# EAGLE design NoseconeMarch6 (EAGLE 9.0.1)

## Sheet 1 of 3: Board to Board Headers
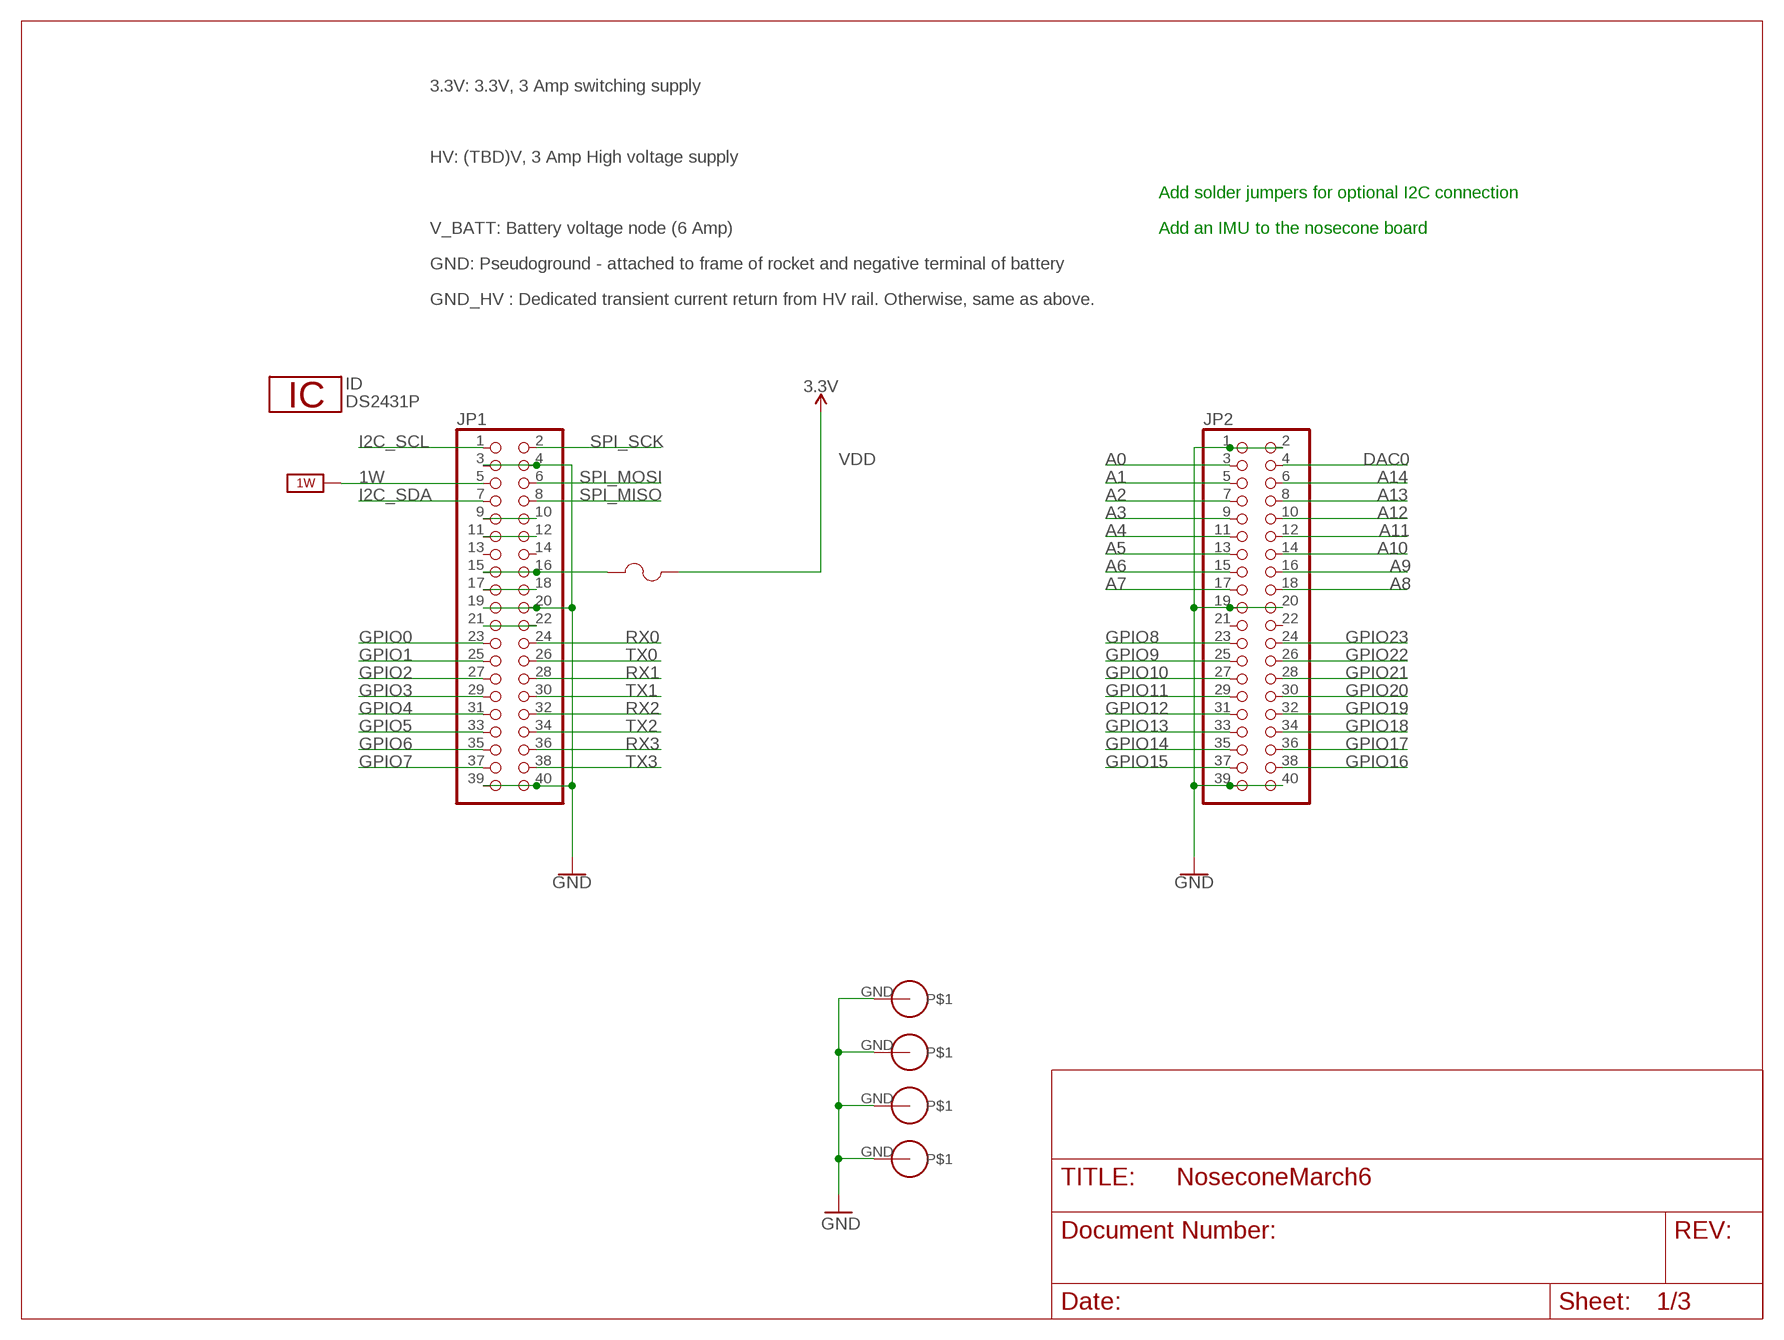
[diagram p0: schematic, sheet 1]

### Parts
F3  0603SFF150F/32-2  [FUS0603_TYCO]
ID  DS2431P  [TSOC6]
JP1  PINHD-2X20  [2X20]
JP2  PINHD-2X20  [2X20]
U$1  PS/104-MOUNTING-HOLE  [PC/104-MOUNTING-HOLE]
U$2  PS/104-MOUNTING-HOLE  [PC/104-MOUNTING-HOLE]
U$3  PS/104-MOUNTING-HOLE  [PC/104-MOUNTING-HOLE]
U$4  PS/104-MOUNTING-HOLE  [PC/104-MOUNTING-HOLE]

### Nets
1W: JP1.5 ; supply symbol labelled 1W_SUP
A0: JP2.3
A1: JP2.5
A2: JP2.7
A3: JP2.9
A4: JP2.11
A5: JP2.13
A6: JP2.15
A7: JP2.17
A8: JP2.18
A9: JP2.16
A10: JP2.14
A11: JP2.12
A12: JP2.10
A13: JP2.8
A14: JP2.6
DAC0: JP2.4
GND: JP1.3 JP1.4 JP1.19 JP1.20 JP1.39 JP1.40 JP2.1 JP2.2 JP2.19 JP2.20 JP2.39 JP2.40 U$1.GND U$2.GND U$3.GND U$4.GND ; also sheet 2,3
GND_HV: JP1.21 JP1.22
GPIO0: JP1.23 ; also sheet 3
GPIO1: JP1.25 ; also sheet 3
GPIO2: JP1.27
GPIO3: JP1.29
GPIO4: JP1.31 ; also sheet 3
GPIO5: JP1.33 ; also sheet 3
GPIO6: JP1.35 ; also sheet 2
GPIO7: JP1.37 ; also sheet 2
GPIO8: JP2.23
GPIO9: JP2.25
GPIO10: JP2.27
GPIO11: JP2.29
GPIO12: JP2.31
GPIO13: JP2.33
GPIO14: JP2.35
GPIO15: JP2.37
GPIO16: JP2.38
GPIO17: JP2.36
GPIO18: JP2.34
GPIO19: JP2.32
GPIO20: JP2.30
GPIO21: JP2.28
GPIO22: JP2.26 ; also sheet 2
GPIO23: JP2.24 ; also sheet 2
I2C_SCL: JP1.1 ; also sheet 2,3
I2C_SDA: JP1.7 ; also sheet 2,3
N$1: JP1.17 JP1.18
N$2: JP1.11 JP1.12
N$3: F3.1 JP1.15 JP1.16
N$4: JP1.9 JP1.10
RX0: JP1.24
RX1: JP1.28
RX2: JP1.32 ; also sheet 2
RX3: JP1.36 ; also sheet 2
SPI_MISO: JP1.8 ; also sheet 2,3
SPI_MOSI: JP1.6 ; also sheet 2,3
SPI_SCK: JP1.2 ; also sheet 2,3
TX0: JP1.26
TX1: JP1.30
TX2: JP1.34 ; also sheet 2
TX3: JP1.38 ; also sheet 2
VDD: F3.2 ; supply symbol labelled 3.3V ; also sheet 2,3
Unconnected: JP1.13 JP1.14 JP2.21 JP2.22

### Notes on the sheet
- 3.3V: 3.3V, 3 Amp switching supply
- HV: (TBD)V, 3 Amp High voltage supply
- Add solder jumpers for optional I2C connection
- V_BATT: Battery voltage node (6 Amp) | Add an IMU to the nosecone board
- GND: Pseudoground - attached to frame of rocket and negative terminal of battery
- GND_HV : Dedicated transient current return from HV rail. Otherwise, same as above.

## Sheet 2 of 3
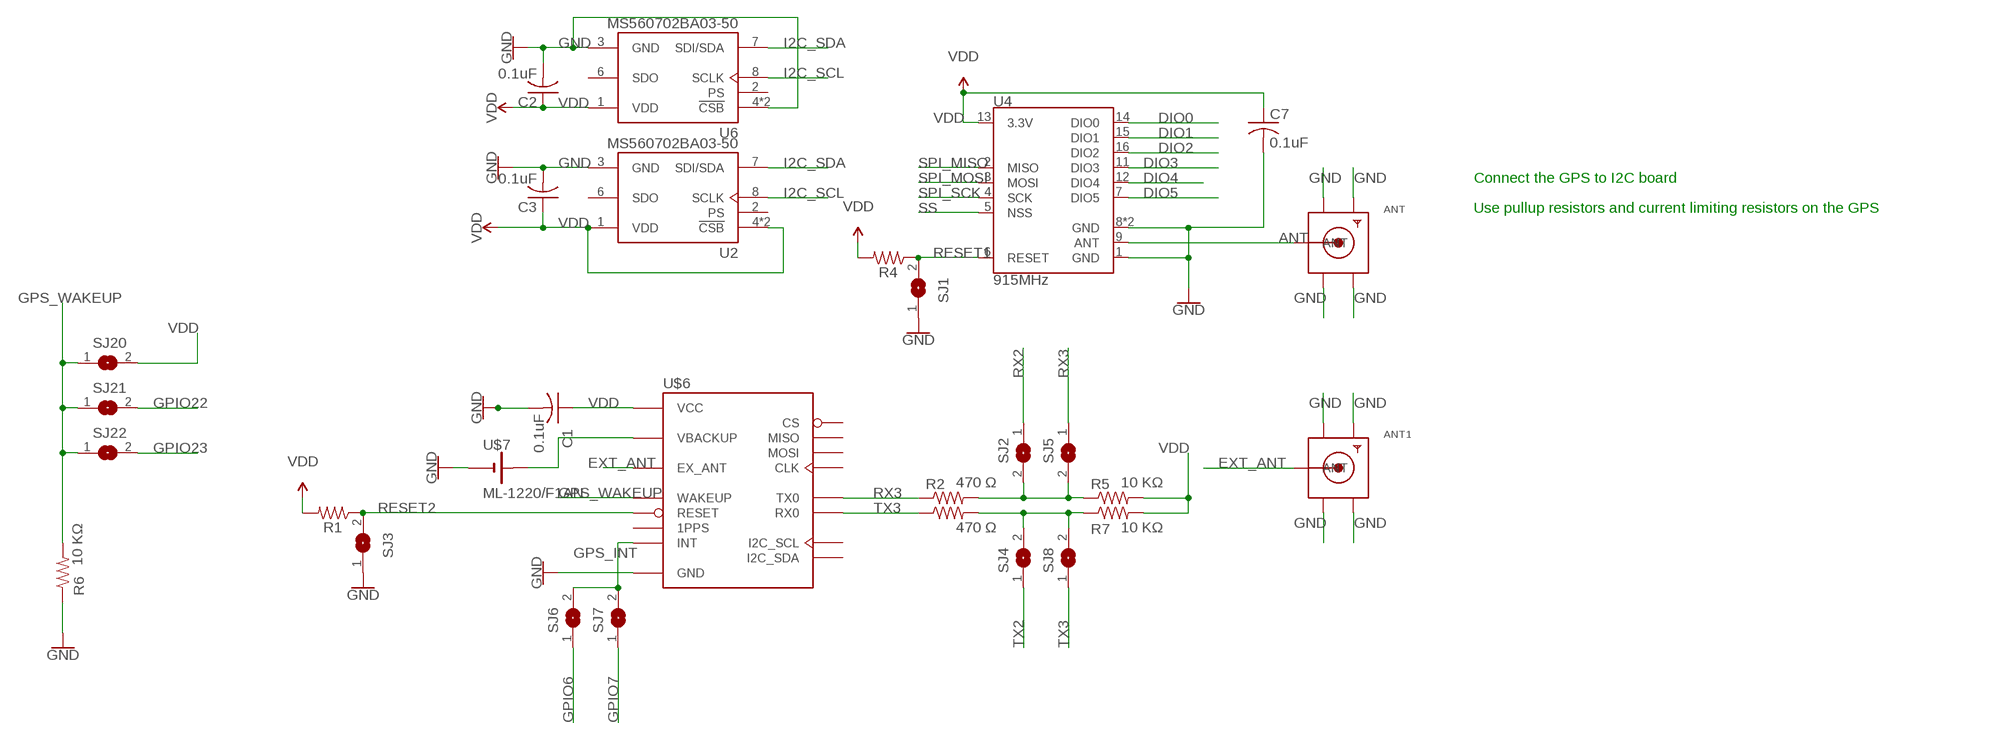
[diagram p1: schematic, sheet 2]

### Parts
ANT  SMACONNECTOR_EDGE  [SMA_EDGELAUNCH]
ANT1  SMACONNECTOR_EDGE  [SMA_EDGELAUNCH]
C1  0.1uF  C-USC0805  [C0805]
C2  0.1uF  C-USC0805  [C0805]
C3  0.1uF  C-USC0805  [C0805]
C7  0.1uF  C-USC0805  [C0805]
R1  330  R-US_R1206  [R1206]
R2  470 Ω  R-US_R1206  [R1206]
R3  470 Ω  R-US_R1206  [R1206]
R4  330  R-US_R1206  [R1206]
R5  10 KΩ  R-US_R1206  [R1206]
R6  10 KΩ  R-US_R1206  [R1206]
R7  10 KΩ  R-US_R1206  [R1206]
SJ1  SJ  [SJ]
SJ2  SJ  [SJ]
SJ3  SJ  [SJ]
SJ4  SJ  [SJ]
SJ5  SJ  [SJ]
SJ6  SJ  [SJ]
SJ7  SJ  [SJ]
SJ8  SJ  [SJ]
SJ20  SJ  [SJ]
SJ21  SJ  [SJ]
SJ22  SJ  [SJ]
U2  MS560702BA03-50  [SON125P300X500X100-8N]
U4  915MHz  RFM69HCW-915  [RFM69HCW-XXXS2]
U6  MS560702BA03-50  [SON125P300X500X100-8N]
U$6  XA1110  [XA1110]
U$7  ML-1220/F1AN  [ML-1220/F1AN]

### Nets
ANT: ANT.P(ANT) U4.9(ANT)
DIO0: U4.14(DIO0)
DIO1: U4.15(DIO1)
DIO2: U4.16(DIO2)
DIO3: U4.11(DIO3)
DIO4: U4.12(DIO4)
DIO5: U4.7(DIO5)
EXT_ANT: ANT1.P(ANT) U$6.P$2(EX_ANT)
GND: ANT1.GND@1(GND4) ANT1.GND@2(GND3) ANT1.GND@3(GND2) ANT1.GND@4(GND1) ANT.GND@1(GND4) ANT.GND@2(GND3) ANT.GND@3(GND2) ANT.GND@4(GND1) C2.2 C3.2 C7.2 R6.1 SJ1.1 SJ3.1 U2.3(GND) U4.1(GND) U4.8(GND) U4.10(GND) U6.3(GND) U6.4(!CSB) U6.5(!CSB) U$6.P$1(GND) U$6.P$3(GND) U$6.P$4(GND) U$6.P$5(GND) U$6.P$6(GND) U$6.P$9(GND) U$6.P$10(GND) U$6.P$11(GND) U$6.P$24(GND) ; also sheet 1,3
GPIO6: SJ6.1 ; also sheet 1
GPIO7: SJ7.1 ; also sheet 1
GPIO22: SJ21.2 ; also sheet 1
GPIO23: SJ22.2 ; also sheet 1
GPS_INT: SJ6.2 SJ7.2 U$6.P$16(INT)
GPS_RX: R3.2 R7.1 SJ4.2 SJ8.2
GPS_TX: R2.2 R5.1 SJ2.2 SJ5.2
GPS_WAKEUP: R6.2 SJ20.1 SJ21.1 SJ22.1 U$6.P$12(WAKEUP)
I2C_SCL: U2.8(SCLK) U6.8(SCLK) ; also sheet 1,3
I2C_SDA: U2.7(SDI/SDA) U6.7(SDI/SDA) ; also sheet 1,3
N$5: U$7.NEG(N) ; supply symbol labelled GND
N$6: C1.2
RESET1: R4.1 SJ1.2 U4.6(RESET)
RESET2: R1.1 SJ3.2 U$6.P$22(RESET)
RX2: SJ2.1 ; also sheet 1
RX3: R2.1 SJ5.1 U$6.P$19(TX0) ; also sheet 1
SPI_MISO: U4.2(MISO) ; also sheet 1,3
SPI_MOSI: U4.3(MOSI) ; also sheet 1,3
SPI_SCK: U4.4(SCK) ; also sheet 1,3
SS: U4.5(NSS)
TX2: SJ4.1 ; also sheet 1
TX3: R3.1 SJ8.1 U$6.P$20(RX0) ; also sheet 1
VBACKUP: U$6.P$8(VBACKUP) U$7.POS(P)
VDD: C1.1 C2.1 C3.1 C7.1 R1.2 R4.2 R5.2 R7.2 SJ20.2 U2.1(VDD) U2.4(!CSB) U2.5(!CSB) U4.13(3.3V) U6.1(VDD) U$6.P$7(VCC) ; also sheet 1,3
Unconnected: U2.2(PS) U2.6(SDO) U6.2(PS) U6.6(SDO) U$6.P$13(I2C_SDA) U$6.P$14(I2C_SCL) U$6.P$15(MISO) U$6.P$17(MOSI) U$6.P$18(CLK) U$6.P$21(1PPS) U$6.P$23(CS)

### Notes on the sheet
- Connect the GPS to I2C board
- Use pullup resistors and current limiting resistors on the GPS

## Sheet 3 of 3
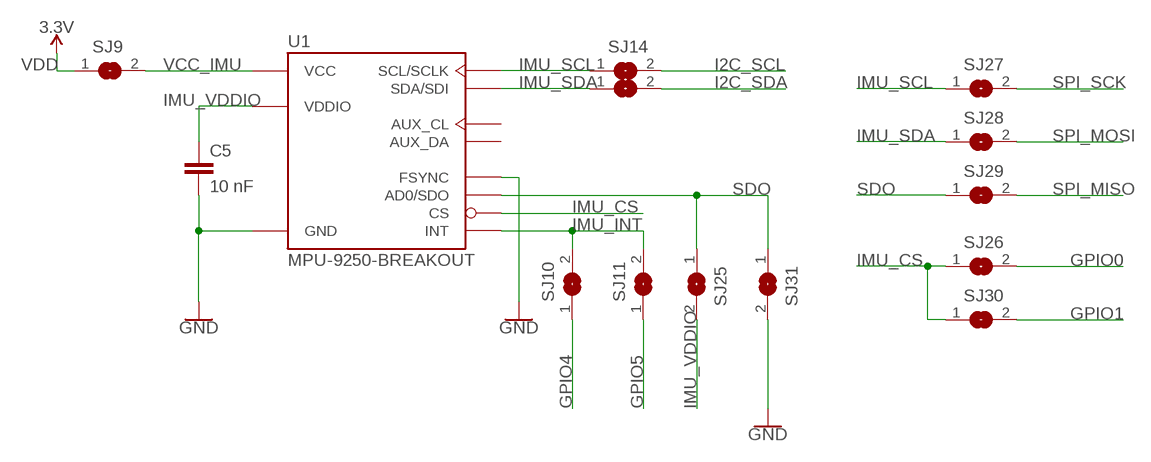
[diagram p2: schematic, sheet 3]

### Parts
C5  10 nF  C-EUC0805  [C0805]
SJ9  SJ  [SJ]
SJ10  SJ  [SJ]
SJ11  SJ  [SJ]
SJ14  SJ  [SJ]
SJ15  SJ  [SJ]
SJ25  SJ  [SJ]
SJ26  SJ  [SJ]
SJ27  SJ  [SJ]
SJ28  SJ  [SJ]
SJ29  SJ  [SJ]
SJ30  SJ  [SJ]
SJ31  SJ  [SJ]
U1  MPU-9250-BREAKOUT  [MPU-9250-BREAKOUT]

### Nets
GND: C5.2 SJ31.2 U1.FSYNC U1.GND ; also sheet 1,2
GPIO0: SJ26.2 ; also sheet 1
GPIO1: SJ30.2 ; also sheet 1
GPIO4: SJ10.1 ; also sheet 1
GPIO5: SJ11.1 ; also sheet 1
I2C_SCL: SJ14.2 ; also sheet 1,2
I2C_SDA: SJ15.2 ; also sheet 1,2
IMU_CS: SJ26.1 SJ30.1 U1.NCS(CS)
IMU_INT: SJ10.2 SJ11.2 U1.INT
IMU_SCL: SJ14.1 SJ27.1 U1.SCL/SCLK
IMU_SDA: SJ15.1 SJ28.1 U1.SDA/SDI
IMU_VDDIO: C5.1 SJ25.2 U1.VDDIO
SDO: SJ25.1 SJ29.1 SJ31.1 U1.AD0/SDO
SPI_MISO: SJ29.2 ; also sheet 1,2
SPI_MOSI: SJ28.2 ; also sheet 1,2
SPI_SCK: SJ27.2 ; also sheet 1,2
VCC_IMU: SJ9.2 U1.VDD(VCC)
VDD: SJ9.1 ; supply symbol labelled 3.3V ; also sheet 1,2
Unconnected: U1.AUX_CL U1.AUX_DA

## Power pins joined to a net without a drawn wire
1W: ID.2(1W)
GND: ID.1(GND)

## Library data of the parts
ANT ANT1 = adafruit:SMACONNECTOR: SMA Connector 90° DIP SMA Connector, 50 Ohm (4UConnector: 07259)
C1-C3 C7 = rcl:C-US: CAPACITOR, American symbol; SPICEPREFIX: C
C5 = rcl:C-EU: CAPACITOR, European symbol; SPICEPREFIX: C
F3 = CU inSpace 2019 Parts:0603SFF150F/32-2; MANUFACTURER_PART_NUMBER: 0603SFF150F322; VENDOR: Littelfuse Inc
ID = 1wire:DS2431: 1024-Bit EEPROM
JP1 JP2 = pinhead:PINHD-2X20: PIN HEADER
R1-R7 = rcl:R-US_: RESISTOR, American symbol; SPICEPREFIX: R
SJ1-SJ11 SJ14 SJ15 SJ20-SJ22 SJ25-SJ31 = jumper:SJ: SMD solder JUMPER
U1 = Sensors Board:MPU-9250-BREAKOUT
U2 U6 = MS560702BA03-50:MS560702BA03-50: BAROMETRIC PRESSURE SENSOR; AVAILABILITY: Unavailable; DESCRIPTION: MS5607-02BA03 Series 3 V 1 to 120 kPa Absolute Barometric Pressure Sensor; EU_ROHS_COMPLIANCE: Compliant; LINK: http://www.te.com/usa-en/product-MS560702BA03-50.html; MF: TE Connectivity; MP: MS560702BA03-50; PACKAGE: SMD-8 TE Connectivity; PRICE: None
U4 = SparkFun-RF:RFM69H: Hope RF RFM69H ISM Transceiver Module The RFM69H is a transceiver module capable of operation over a wide frequency range, including the 315,433,868 and 915MHz license-free ISM (Industry Scientific and Medical) frequency bands. All major RF communication parameters are programmable and most of them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; PROD_ID: IC-11997
U$1-U$4 = CU inSpace 2019 Parts:PS/104-MOUNTING-HOLE: Mounting hole for PC/104 board.
U$6 = Sensors Board:XA1110
U$7 = Sensors Board:ML-1220/F1AN

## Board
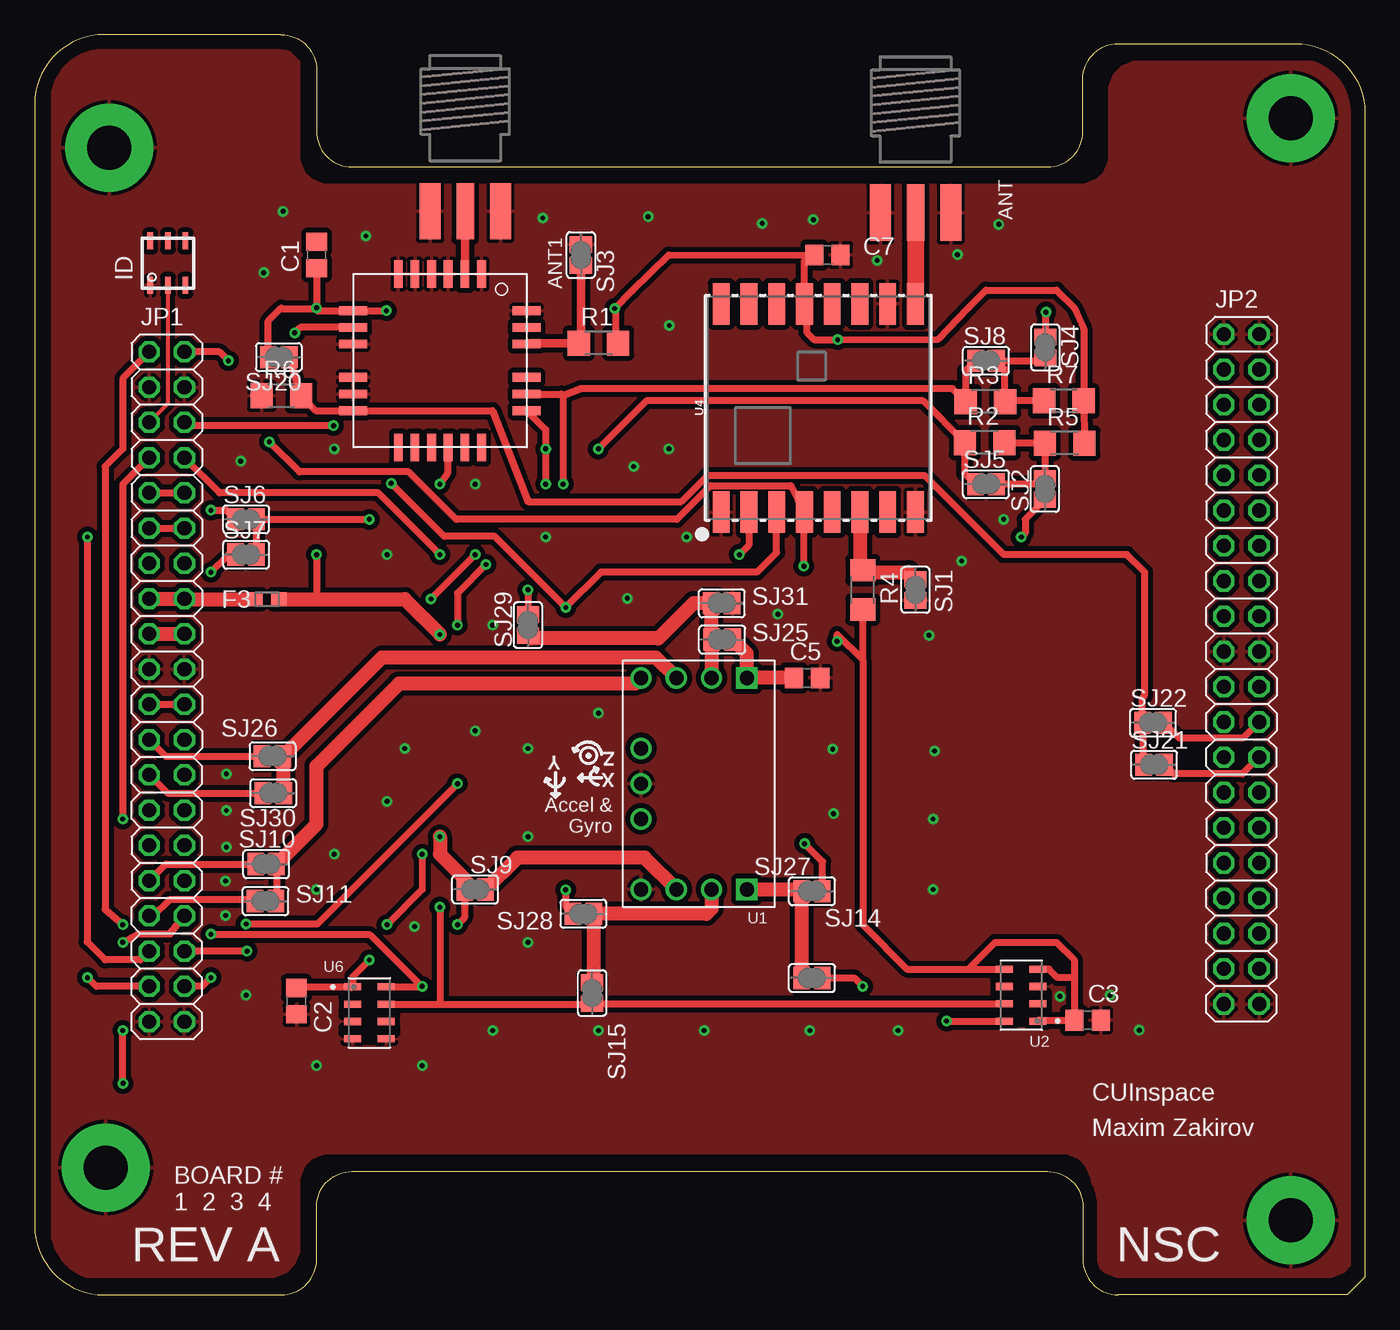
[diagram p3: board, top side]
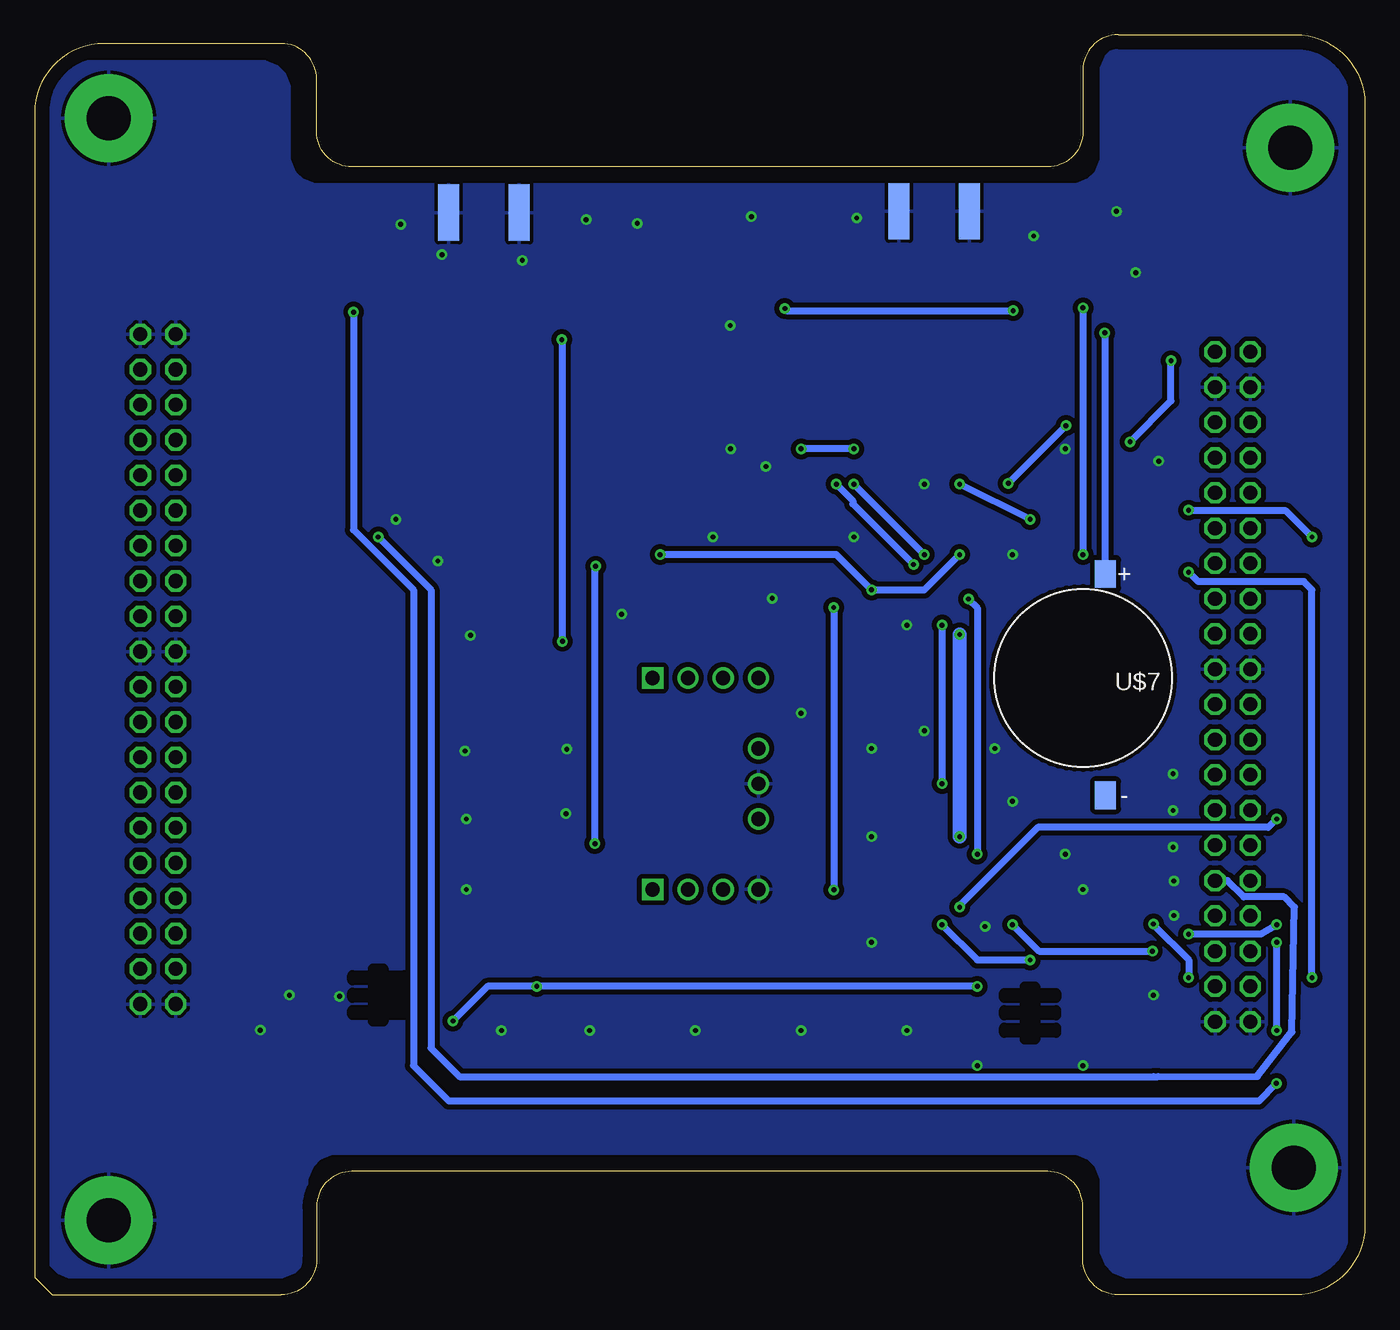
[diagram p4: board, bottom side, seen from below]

Size 95.89 x 90.81 mm. Coordinates in mm from the lower left corner, seen from the top.
Outline: 0,85.81 0,5 arc90 5,0 17.78,0 arc90 20.32,2.54 20.32,6.35 arc-90 22.86,8.89 73.03,8.89 arc-90 75.56,6.35 75.56,2.54 arc90 78.11,0 94.61,0 95.89,1.27 95.89,85.17 arc90 90.89,90.17 78.11,90.17 arc90 75.56,87.63 75.56,83.82 arc-90 73.03,81.28 22.86,81.28 arc-90 20.32,83.82 20.32,88.27 arc90 17.78,90.81 5,90.81 arc90 0,85.81
Copper layers (1*16): Top 0.035mm / dielectric 1.5mm / Bottom 0.035mm
Design rules "default": minimum track width 6mil, minimum drill 0.35mm, track to track 6mil, track to pad 6mil, pad to pad 6mil, via to via 6mil, smd to smd 6mil, copper to edge 40mil, drill to drill 6mil, minimum pad ring 10mil, minimum via ring 8mil, stop-mask expansion 4mil, vias tented up to drill 0mil, thermal gap 10mil

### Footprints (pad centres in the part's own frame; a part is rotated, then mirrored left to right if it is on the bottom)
SMA_EDGELAUNCH = smd 4.064 x 1.524: GND@1 2.032,-2.54; GND@2 2.032,2.54 | smd 4.064 x 1.524 bottom: GND@3 2.032,2.54; GND@4 2.032,-2.54 | smd 4.064 x 1.27: P 2.032,0
C0805 = smd 1.3 x 1.5: 1 -0.95,0; 2 0.95,0
FUS0603_TYCO = smd 1.092 x 0.991: 1 -0.851,0; 2 0.851,0
TSOC6 = smd 0.406 x 1.219: 1 -1.27,-1.6; 2 0,-1.6; 3 1.27,-1.6; 4 1.27,1.6; 5 0,1.6; 6 -1.27,1.6
2X20 = drill 1.016 octagon: 1 -24.13,-1.27; 2 -24.13,1.27; 3 -21.59,-1.27; 4 -21.59,1.27; 5 -19.05,-1.27; 6 -19.05,1.27; 7 -16.51,-1.27; 8 -16.51,1.27; 9 -13.97,-1.27; 10 -13.97,1.27; 11 -11.43,-1.27; 12 -11.43,1.27; 13 -8.89,-1.27; 14 -8.89,1.27; 15 -6.35,-1.27; 16 -6.35,1.27; 17 -3.81,-1.27; 18 -3.81,1.27; 19 -1.27,-1.27; 20 -1.27,1.27; 21 1.27,-1.27; 22 1.27,1.27; 23 3.81,-1.27; 24 3.81,1.27; 25 6.35,-1.27; 26 6.35,1.27; 27 8.89,-1.27; 28 8.89,1.27; 29 11.43,-1.27; 30 11.43,1.27; 31 13.97,-1.27; 32 13.97,1.27; 33 16.51,-1.27; 34 16.51,1.27; 35 19.05,-1.27; 36 19.05,1.27; 37 21.59,-1.27; 38 21.59,1.27; 39 24.13,-1.27; 40 24.13,1.27
R1206 = smd 1.6 x 1.803: 1 -1.422,0; 2 1.422,0
SJ = smd 1.168 x 1.6: 1 -0.762,0; 2 0.762,0
MPU-9250-BREAKOUT = drill 1.016: AD0/SDO -0.533,-7.62; AUX_CL 4.547,-2.54; AUX_DA 4.547,2.54; FSYNC 4.547,0; GND 4.547,7.62; INT 4.547,-7.62; NCS 2.007,-7.62; SDA/SDI -0.533,7.62; VDD 2.007,7.62 | drill 1.016 square: SCL/SCLK -3.073,7.62; VDDIO -3.073,-7.62
SON125P300X500X100-8N = smd 1.31 x 0.53: 1 -1.2,1.875; 2 -1.2,0.625; 3 -1.2,-0.625; 4 -1.2,-1.875; 5 1.2,-1.875; 6 1.2,-0.625; 7 1.2,0.625; 8 1.2,1.875
RFM69HCW-XXXS2 = smd 3 x 1.2: 1 -7.5,7; 2 -7.5,5; 3 -7.5,3; 4 -7.5,1; 5 -7.5,-1; 6 -7.5,-3; 7 -7.5,-5; 8 -7.5,-7; 9 7.5,-7; 10 7.5,-5; 11 7.5,-3; 12 7.5,-1; 13 7.5,1; 14 7.5,3; 15 7.5,5; 16 7.5,7
PC/104-MOUNTING-HOLE = drill 3.175 pad 6.35: GND 0,0
XA1110 = smd 2 x 0.635: P$1 -6.25,3; P$2 -6.25,1.8; P$3 -6.25,0.6; P$4 -6.25,-0.6; P$5 -6.25,-1.8; P$6 -6.25,-3; P$13 6.25,-3; P$14 6.25,-1.8; P$15 6.25,-0.6; P$16 6.25,0.6; P$17 6.25,1.8; P$18 6.25,3 | smd 0.635 x 2: P$7 -3.6,-6.25; P$8 -2.4,-6.25; P$9 -1.2,-6.25; P$10 1.2,-6.25; P$11 2.4,-6.25; P$12 3.6,-6.25; P$19 3.6,6.25; P$20 2.4,6.25; P$21 1.2,6.25; P$22 -1.2,6.25; P$23 -2.4,6.25; P$24 -3.6,6.25
ML-1220/F1AN = smd 1.5 x 2: NEG -1.625,8.45; POS -1.625,-7.5

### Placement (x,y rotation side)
ANT  63.5,80.01 270 top
ANT1  31.04,80.11 270 top
C1  20.32,74.93 90 top
C2  18.87,21.16 270 top
C3  75.9,19.79 0 top
C5  55.68,44.45 0 top
C7  57.15,74.93 0 top
F3  16.75,50.13 0 top
ID  9.6,74.35 0 top
JP1  9.53,43.81 270 top
JP2  87,45.09 270 top
R1  40.64,68.58 0 top
R2  68.48,61.42 0 top
R3  68.53,64.36 0 top
R4  59.69,50.8 270 top
R5  74.24,61.37 0 top
R6  17.78,64.77 0 top
R7  74.19,64.41 0 top
SJ1  63.5,50.8 90 top
SJ2  72.82,58.06 90 top
SJ3  39.37,74.93 270 top
SJ4  72.85,68.28 270 top
SJ5  68.58,58.42 0 top
SJ6  15.24,55.88 0 top
SJ7  15.24,53.34 0 top
SJ8  68.58,67.31 0 top
SJ9  31.75,29.21 0 top
SJ10  16.69,31.04 0 top
SJ11  16.64,28.37 0 top
SJ14  56.03,22.83 0 top
SJ15  40.18,21.74 270 top
SJ20  17.6,67.56 180 top
SJ21  80.7,38.2 0 top
SJ22  80.62,41.22 0 top
SJ25  49.56,47.22 0 top
SJ26  17.14,38.81 180 top
SJ27  56.03,29.08 0 top
SJ28  39.55,27.46 180 top
SJ29  35.56,48.26 90 top
SJ30  17.2,36.14 180 top
SJ31  49.53,49.83 0 top
U1  48.26,36.83 180 top
U2  71.12,21.59 180 top
U4  56.49,63.91 90 top
U6  24.13,20.32 0 top
U$1  5.36,82.65 0 top
U$2  90.55,84.79 0 top
U$3  5.13,9.17 0 top
U$4  90.55,5.36 0 top
U$6  29.21,67.31 270 top
U$7  20.32,44.45 180 bottom

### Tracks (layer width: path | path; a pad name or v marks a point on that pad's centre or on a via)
1W
  Top 0.305: ID.2 9.6,64.21 JP1.5
ANT
  Top 1.219: U4.9 ANT.P
EXT_ANT
  Top 0.61: U$6.P$2 31.01,78.05 ANT1.P
GND  (via drill 0.35)
  other vias: 16.51,73.66 23.88,76.3 17.91,78.08 36.63,77.6 44.22,77.7 52.45,77.22 45.75,69.85 56.13,77.47 60.73,74.55 66.52,74.96 69.49,77.14 66.83,52.88 64.47,47.52 64.87,39.19 27.38,26.54 14.86,60.07 53.57,49.05 42.72,50.19 35.56,39.37 40.64,41.91 31.75,40.64 35.56,33.02 26.67,39.37 25.4,35.56 13.82,37.54 13.82,34.9 13.77,29.82 13.77,27.33 21.59,31.75 20.32,29.21 15.24,21.59 13.82,32.26 20.32,16.51 27.94,16.51 33.02,19.05 40.64,19.05 35.56,25.4 48.26,19.05 55.88,19.05 62.23,19.05 64.77,29.21 64.77,34.29 57.58,34.67 57.53,39.32 73.91,21.51 77.52,21.59 79.63,19.08 46.99,54.61 33.02,48.26 31.75,58.42 43.18,59.69 45.72,60.96 69.85,55.88 25.4,53.34 36.83,54.61 21.59,60.96
  pour Top (isolate 0.356): 1.27,87.63 1.27,88.9 2.54,90.17 17.25,90.17 18.15,89.8 19.05,88.9 19.05,81.81 19.42,80.91 19.95,80.38 20.85,80.01 41.91,80.01 75.67,80.01 76.57,80.38 77.1,80.91 77.47,81.81 77.47,87.1 77.84,88 78.37,88.53 79.27,88.9 93.45,88.9 94.35,88.53 94.88,88 95.25,87.1 95.25,36.83 95.25,3.07 94.88,2.17 94.35,1.64 93.45,1.27 78.74,1.27 78,1.27 77.1,1.64 76.57,2.17 76.2,3.07 76.2,8.36 75.83,9.26 75.3,9.79 74.4,10.16 20.85,10.16 19.95,9.79 19.42,9.26 19.05,8.36 19.05,3.07 18.68,2.17 18.15,1.64 17.25,1.27 6.35,1.27 5.08,1.27 3.07,1.27 2.17,1.64 1.64,2.17 1.27,3.07 1.27,8.89
  pour Bottom (isolate 0.356): 1.27,88.9 2.17,89.8 3.07,90.17 17.25,90.17 18.15,89.8 18.68,89.27 19.05,88.37 19.05,81.81 19.42,80.91 19.95,80.38 20.85,80.01 75.67,80.01 76.57,80.38 77.1,80.91 77.47,81.81 77.47,87.1 77.84,88 78.37,88.53 79.27,88.9 93.45,88.9 94.35,88.53 94.88,88 95.25,87.1 95.25,3.13 94.88,2.23 94.24,1.59 93.45,1.27 78,1.27 77.1,1.64 76.57,2.17 76.2,3.07 76.2,8.36 75.83,9.26 75.3,9.79 74.4,10.16 20.85,10.16 19.95,9.79 19.42,9.26 19.05,8.36 19.05,3.07 18.68,2.17 18.15,1.64 17.25,1.27 3.07,1.27 2.17,1.64 1.64,2.17 1.27,3.07
GND_HV
  Top 0.508: JP1.21 JP1.22
GPIO0
  Top 0.508: JP1.23 9.47,38.79 16.36,38.79 SJ26.2
GPIO1
  Top 0.508: JP1.25 9.58,36.14 SJ30.2
GPIO4
  Top 0.508: JP1.31 9.45,31.04 SJ10.1
GPIO5
  Top 0.508: JP1.33 8.56,27.3 9.73,28.47 15.77,28.47 SJ11.1
GPIO6  (via drill 0.35)
  Top 0.508: JP1.35 7.62,24.13 5.08,24.13 3.79,25.43 3.79,54.59 v3.81,54.61 | v12.7,56.54 13.82,56.54 SJ6.1
  Bottom 0.508: v3.81,54.61 5.69,56.49 12.7,56.49 v12.7,56.54
GPIO7  (via drill 0.35)
  Top 0.508: JP1.37 4.45,22.23 v3.81,22.86 | v12.7,52.07 13.97,53.34 SJ7.1
  Bottom 0.508: v3.81,22.86 3.81,50.8 4.39,51.38 12.01,51.38 v12.7,52.07
GPIO22
  Top 0.508: JP2.26 87.07,37.54 82.12,37.54 SJ21.2
GPIO23
  Top 0.508: JP2.24 87.1,40.11 82.5,40.11 SJ22.2
GPS_INT  (via drill 0.35)
  Top 0.508: SJ7.2 SJ6.2 v24.13,55.88 | v29.21,58.42 29.79,59.23 U$6.P$16
  Bottom 0.508: v24.13,55.88 v29.21,58.42
GPS_RX
  Top 0.508: R7.1 70,64.41 R3.2 69.95,66.7 SJ8.2 72.64,67.31 SJ4.2 72.77,67.44
GPS_TX
  Top 0.508: R2.2 72.77,61.42 R5.1 | SJ5.2 72.42,58.42 SJ2.2 R5.1 | R5.1
GPS_WAKEUP
  Top 0.508: SJ21.1 79.93,41.15 SJ22.1 79.86,43.03 80.01,43.18 80.01,52.07 78.74,53.34 69.85,53.34 64.16,59.03 48.5,59.03 46.62,57.15 35.56,57.15 33,63.71 U$6.P$12 20.26,63.71 R6.2 SJ20.1
I2C_SCL  (via drill 0.35)
  Top 0.508: JP1.1 6.35,66.04 6.35,60.96 5.08,59.69 5.08,27.76 v6.35,26.67 | U6.8 27.91,22.2 | 27.91,22.2 v27.94,22.23 | v65.73,19.74 65.76,19.71 U2.8 | SJ14.2 59.08,22.84 v59.69,22.23 | 27.91,22.2 24.17,25.93 12.75,25.93 v12.7,25.98
  Bottom 0.508: v27.94,22.23 v59.69,22.23 63.25,22.23 v65.73,19.74 | v6.35,26.67 7.49,25.98 v12.7,25.98
I2C_SDA  (via drill 0.35)
  Top 0.508: U2.7 69.89,20.98 SJ15.2 40.15,20.95 29.21,20.95 | JP1.7 6.35,58.42 v6.35,34.29 | U6.7 29.21,20.95 | v29.21,27.94 29.21,20.95
  Bottom 0.508: v6.35,34.29 6.96,33.68 23.57,33.68 29.16,28.09 29.16,27.99 v29.21,27.94
IMU_CS
  Top 1.016: U1.NCS 44.78,45.92 25.02,45.92 SJ26.1 17.91,36.2 SJ30.1
IMU_INT
  Top 0.508: SJ10.2 17.45,28.42 SJ11.2
  Top 1.016: SJ10.2 20.32,33.91 20.32,38.1 26.26,44.04 43.31,44.04 U1.INT
IMU_SCL
  Top 1.016: 51.44,29.21 U1.SCL/SCLK 55.14,29.21 SJ27.1 SJ14.1
IMU_SDA
  Top 1.016: 40.31,27.51 SJ28.1 | 40.23,22.55 SJ15.1 40.31,22.63 SJ28.1 | SJ28.1 48.41,27.46 48.79,27.84 U1.SDA/SDI
IMU_VDDIO
  Top 1.016: C5.1 U1.VDDIO 51.33,46.2 SJ25.2
N$1
  Top 1.016: JP1.17 JP1.18
N$2
  Top 0.508: JP1.11 JP1.12
N$3
  Top 1.016: JP1.15 JP1.16 10.79,50.13 F3.1
N$4
  Top 0.508: JP1.9 JP1.10
RESET1
  Top 1.016: U4.6 59.49,52.42 | R4.1 59.84,52.07 62.99,52.07 SJ1.2
  Top 1.219: 59.49,52.42 R4.1
RESET2
  Top 0.61: U$6.P$22 35.53,68.58 R1.1 39.37,68.73 SJ3.2
RX2  (via drill 0.35)
  Top 0.508: SJ2.1 71.4,55.88 71.4,54.89 v71.12,54.61
  Bottom 0.508: v71.12,54.61 67.31,50.8 67.31,17.78 65.25,15.72 15.24,15.72 | 15.24,15.72 14.91,15.72 | 15.24,15.72 7.75,15.75 5.26,18.95 5.08,27.94 5.82,28.68 8.74,28.68 9.91,29.84 JP1.32
RX3  (via drill 0.35)
  Top 0.508: U$6.P$19 36.83,62.34 v36.83,60.96 v36.83,58.42 | v31.75,53.34 28.57,50.16 v28.57,50.14 | v27.94,31.75 27.94,29.21 v25.4,26.67 | v15.32,24.77 JP1.36 | v40.64,60.96 44.09,64.41 64.06,64.41 R2.1 67.06,59.18 SJ5.1
  Bottom 0.508: v36.83,58.42 v31.75,53.34 | v28.57,50.14 27.94,49.51 v27.94,31.75 | v25.4,26.67 23.5,24.77 v15.32,24.77 | v36.83,60.96 v40.64,60.96
SDO
  Top 1.016: SJ29.1 35.76,47.3 44.96,47.3 47.5,49.84 SJ31.1 48.77,47.24 SJ25.1 U1.AD0/SDO
SPI_MISO  (via drill 0.35)
  Top 0.508: U4.2 51.49,54.03 v50.8,53.34 | JP1.8 13.34,57.78 24.77,57.78 v29.21,53.34 | v35.56,50.8 SJ29.2
  Bottom 0.508: v50.8,53.34 38.1,53.34 v35.56,50.8 31.75,50.8 v29.21,53.34
SPI_MOSI  (via drill 0.35)
  Top 0.508: 53.34,56.26 U4.3 53.49,53.49 52.07,52.07 40.82,52.07 v38.28,49.53 33.15,54.66 29.52,54.66 v25.7,58.47 | v21.54,62.64 11.02,62.64 JP1.6 | v38.28,29.18 38.28,27.96 SJ28.2
  Bottom 0.508: v21.54,62.64 v25.7,58.47 | v38.28,49.53 v38.28,29.19 v38.28,29.18
SPI_SCK  (via drill 0.35)
  Top 0.508: v13.97,67.31 13.34,67.94 JP1.2 | v16.92,61.47 19.09,59.3 26.96,59.3 30.38,55.88 46.29,55.88 48.72,58.31 54.5,58.31 55.45,56.37 | SJ27.2 56.79,31.22 v55.5,32.51 | v55.45,52.5 55.45,56.37 | 55.45,56.37 U4.4
  Bottom 0.508: v16.92,61.47 13.97,64.41 v13.97,67.31 | v55.5,32.51 55.5,52.45 v55.45,52.5
SS
  Top 0.508: 57.15,56.07 U4.5 57.15,56.75
TX2  (via drill 0.35)
  Top 0.508: SJ4.1 72.85,69.52 72.9,69.57 v72.9,70.81 | v6.35,25.4 7.47,26.01 9.78,26.01 JP1.34 | v6.38,15.24 6.35,15.27 v6.35,19.05
  Bottom 0.508: v72.9,70.81 72.9,55.12 68.58,50.8 68.58,16.51 66.04,13.97 7.62,13.97 v6.38,15.24 | v6.35,19.05 v6.35,25.4
TX3  (via drill 0.35)
  Top 0.508: U$6.P$20 37.96,64.91 38.1,64.77 | 38.1,64.77 v38.1,58.42 | v32.54,52.63 30.48,50.57 v30.48,48.26 | v30.48,36.83 20.37,26.72 v15.24,26.72 | v12.7,22.86 12.06,22.23 JP1.38 | SJ8.1 67.11,66.6 R3.1 66.17,65.3 39.37,65.3 38.1,64.77
  Bottom 0.508: v38.1,58.42 36.91,57.23 36.91,57 v32.54,52.63 | v30.48,48.26 v30.48,36.83 | v15.24,26.72 15.24,26.67 12.7,24.13 v12.7,22.86
VBACKUP  (via drill 0.35)
  Top 0.508: U$6.P$8 22.95,69.72 19.15,69.72 v18.75,69.32
  Bottom 0.508: U$7.POS 18.7,69.27 v18.75,69.32
VCC_IMU
  Top 1.016: SJ9.2 34.8,31.5 43.97,31.5 U1.VDD
VDD  (via drill 0.35)
  Top 0.406: U6.1 22.84,22.11 | 19.05,22.11 C2.1
  Top 0.508: 59.69,45.74 R4.2 | C3.1 74.87,19.71 | C1.1 v20.32,71.12 20.27,71.06 | 20.27,71.06 20.42,70.91 U$6.P$7 v25.34,70.91 v25.35,70.92 | v20.32,53.34 20.32,50.13 | v57.84,47.09 57.84,47.6 59.69,45.74 | R1.2 41.86,68.78 41.86,71.02 v41.81,71.07 43.08,72.34 45.72,74.93 56.19,74.91 55.88,74.91 55.49,74.51 U4.13 55.65,71.25 55.65,69.37 56.19,68.83 v57.89,68.83 65.15,68.86 67.31,71.12 68.58,72.39 73.66,72.39 74.93,71.12 75.61,69.6 R7.2 R5.2 | U2.1 72.39,19.79 C3.1 | 67.31,23.46 62.9,23.46 59.69,26.67 59.69,45.74 | 67.31,23.46 U2.5 | 67.31,23.46 69.25,25.4 73.66,25.4 74.93,24.13 74.93,22.86 | 74.93,22.86 74.93,19.8 C3.1 | 74.93,22.86 73.74,22.86 73.13,23.47 73.12,23.46 U2.4 | C2.1 18.96,22.2 U6.1 22.93,22.93 v24.13,24.13 | SJ9.1 30.99,27.18 v30.48,26.67 | SJ20.2 16.84,70.18 17.78,71.12 17.84,71.06 20.27,71.06
  Top 1.016: F3.2 20.32,50.13 26.67,50.13 v29.21,47.59 | 41.91,68.58 R1.2 | 56.19,74.91 56.19,74.92 C7.1 | SJ9.1 30.99,29.97 29.21,31.75 v29.21,33.02
  Bottom 0.508: v20.32,71.12 v20.32,53.34 | v41.81,71.07 41.81,71.02 41.71,70.92 v25.35,70.92 | v57.89,68.83 57.89,47.14 v57.84,47.09 | v30.48,26.67 27.94,24.13 v24.13,24.13
  Bottom 1.016: v29.21,47.59 v29.21,33.02

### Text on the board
tPlace: BOARD # / 1 2 3 4 | REV A | NSC
tNames: CUInspace | Maxim Zakirov
Notes: RF Connectors should go in this notch | Debug connectors should go in this notch | Indicator LEDs should be placed in the bottom corners, filling the avaliable space from left to right

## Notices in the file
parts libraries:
SparkFun-PowerSymbols: Licensing: Creative Commons ShareAlike 4.0 International - https://creativecommons.org/licenses/by-sa/4.0
